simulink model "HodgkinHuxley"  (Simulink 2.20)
settings: Solver=ode45  StartTime=0.0  StopTime=1000  MaxStep=0.1  RelTol=1e-3  AbsTol=1e-6
undefined symbols (not defined in the file or in its folder): sfuny, sfunyst

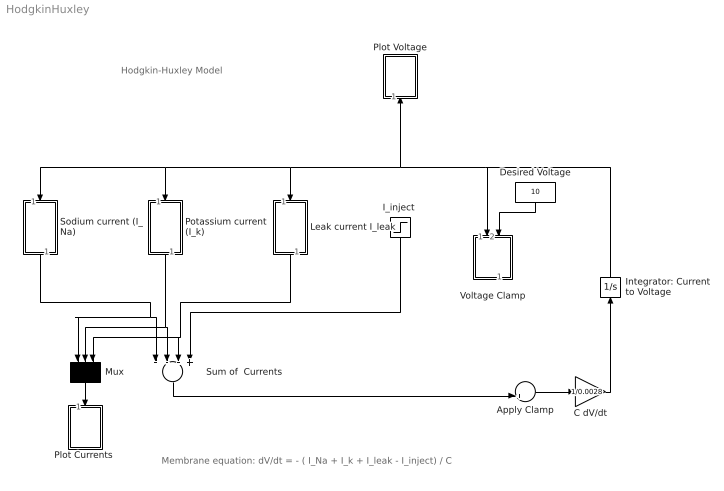
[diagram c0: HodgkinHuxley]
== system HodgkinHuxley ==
  note: Membrane equation: dV/dt = - ( I_Na + I_k + I_leak - I_inject) / C
  note: Hodgkin-Huxley Model
  Apply Clamp : Sum  Inputs=-+
  C dV/dt : Gain  Gain=1/0.0028
  Desired Voltage : Constant  Orientation=down  Value=10
  "I_inject " : Step  Orientation=down  Time=10  Before=0  After=.8
  Integrator: Current to Voltage : Integrator  Orientation=up  ExternalReset=none  InitialConditionSource=internal  InitialCondition=0  LimitOutput=off  UpperSaturationLimit=inf  LowerSaturationLimit=-inf  ShowSaturationPort=off  ShowStatePort=off  AbsoluteTolerance=auto
  Leak current I_leak : Subsystem  Orientation=down
  Mux : Mux  Orientation=down  Inputs=3
  "Plot Currents " : Subsystem  Orientation=down  mask(Storage scope.){}
      mask help: Storage scope using MATLAB graph window. Enter plotting ranges and line type.
      mask init:
      | npts = @4; color = @5; ax = [0, @1, @2, @3]; dt=-1;
  Plot Voltage : Subsystem  Orientation=up  LoadFcn=sfuny([],[],[],'LoadBlock')  StartFcn=sfuny([],[],[],'Start')  StopFcn=sfuny([],[],[],'Stop')  mask(Graph scope.){}
      mask help: Graph scope using MATLAB graph window. Enter plotting ranges and line type.
      mask init:
      | color = @4; ax = [0, @1, @2, @3]; dt = -1;
  Potassium current (I_k) : Subsystem  Orientation=down
  Sodium current (I_Na) : Subsystem  Orientation=down
  Sum of  Currents : Sum  Orientation=down  Inputs=---+
  Voltage Clamp : Subsystem  Orientation=down
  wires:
  Sum of  Currents/1 -> Apply Clamp/2
  Apply Clamp/1 -> C dV/dt/1
  Sodium current (I_Na)/1(I_Na) -> Mux/1, Sum of  Currents/1
  Potassium current (I_k)/1(output Ik) -> Mux/2, Sum of  Currents/2
  Leak current I_leak/1(output  I_leak) -> Mux/3, Sum of  Currents/3
  Mux/1 -> "Plot Currents "/1(x)
  Integrator: Current to Voltage/1 -> Plot Voltage/1(x), Potassium current (I_k)/1(input V), Sodium current (I_Na)/1(input V), Leak current I_leak/1(input V), Voltage Clamp/1(in_1)
  "I_inject "/1 -> Sum of  Currents/4
  Desired Voltage/1 -> Voltage Clamp/2(in_2)
  C dV/dt/1 -> Integrator: Current to Voltage/1

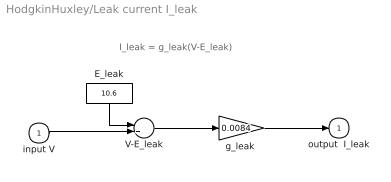
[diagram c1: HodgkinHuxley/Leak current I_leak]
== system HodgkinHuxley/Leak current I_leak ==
  note: I_leak = g_leak(V-E_leak)
  input V : Inport  Port=1  PortWidth=-1  SampleTime=-1
  E_leak : Constant  Orientation=down  Value=10.6
  V-E_leak : Sum  Inputs=-+
  "g_leak " : Gain  Gain=0.0084
  output  I_leak : Outport  Port=1  InitialOutput=0
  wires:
  "g_leak "/1 -> output  I_leak/1
  input V/1 -> V-E_leak/2
  E_leak/1 -> V-E_leak/1
  V-E_leak/1 -> "g_leak "/1

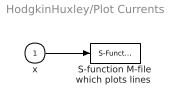
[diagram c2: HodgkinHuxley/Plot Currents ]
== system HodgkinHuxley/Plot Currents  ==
  x : Inport  Port=1  PortWidth=-1  SampleTime=-1
  "S-function M-file which plots lines " : S-Function  LoadFcn=sfunyst([],[],[],'LoadBlock')  FunctionName=sfunyst  Parameters=ax, color, npts, dt  PortCounts=[]  SFunctionModules=''
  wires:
  x/1 -> "S-function M-file which plots lines "/1

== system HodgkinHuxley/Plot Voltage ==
  x : Inport  Port=1  PortWidth=-1  SampleTime=-1
  "S-function M-file which plots lines " : S-Function  FunctionName=sfuny  Parameters=ax, color,dt  PortCounts=[]  SFunctionModules=''
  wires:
  x/1 -> "S-function M-file which plots lines "/1

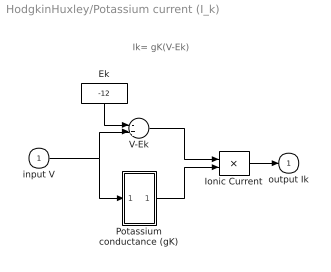
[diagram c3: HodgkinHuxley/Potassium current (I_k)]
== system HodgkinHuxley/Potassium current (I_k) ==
  note: Ik= gK(V-Ek)
  input V : Inport  Port=1  PortWidth=-1  SampleTime=-1
  Ek : Constant  Orientation=down  Value=-12
  Ionic Current : Product  Inputs=2
  Potassium conductance (gK) : Subsystem
  V-Ek : Sum  Inputs=-+
  output Ik : Outport  Port=1  InitialOutput=0
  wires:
  input V/1 -> Potassium conductance (gK)/1(input V), V-Ek/2
  Ionic Current/1 -> output Ik/1
  Ek/1 -> V-Ek/1
  V-Ek/1 -> Ionic Current/1
  Potassium conductance (gK)/1(output gK) -> Ionic Current/2

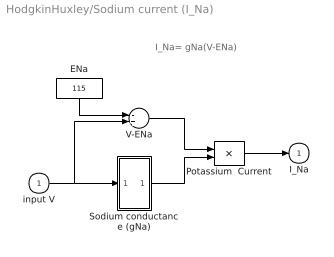
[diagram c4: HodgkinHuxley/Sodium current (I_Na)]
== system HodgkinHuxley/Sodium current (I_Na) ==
  note: I_Na= gNa(V-ENa)
  input V : Inport  Port=1  PortWidth=-1  SampleTime=-1
  ENa : Constant  Orientation=down  Value=115
  Potassium  Current : Product  Inputs=2
  Sodium conductance (gNa) : Subsystem
  V-ENa : Sum  Inputs=-+
  I_Na : Outport  Port=1  InitialOutput=0
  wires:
  input V/1 -> V-ENa/2, Sodium conductance (gNa)/1(input V)
  Potassium  Current/1 -> I_Na/1
  ENa/1 -> V-ENa/1
  V-ENa/1 -> Potassium  Current/1
  Sodium conductance (gNa)/1(ouput gNa) -> Potassium  Current/2

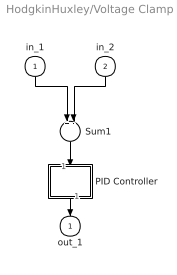
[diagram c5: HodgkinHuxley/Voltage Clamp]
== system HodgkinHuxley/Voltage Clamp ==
  in_1 : Inport  Orientation=down  Port=1  PortWidth=-1  SampleTime=-1
  in_2 : Inport  Orientation=down  Port=2  PortWidth=-1  SampleTime=-1
  PID Controller : Subsystem  Orientation=down  mask(PID Controller){}
      mask help: Enter expressions for proportional, integral, and derivative terms. P+I/s+Ds
      mask init:
      | P=@1; I=@2; D=@3;
  Sum1 : Sum  Orientation=down  Inputs=+-
  out_1 : Outport  Orientation=down  Port=1  InitialOutput=0
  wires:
  PID Controller/1(Out_1) -> out_1/1
  in_2/1 -> Sum1/2
  in_1/1 -> Sum1/1
  Sum1/1 -> PID Controller/1(In_1)

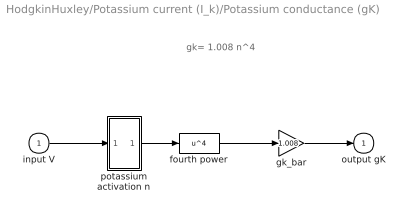
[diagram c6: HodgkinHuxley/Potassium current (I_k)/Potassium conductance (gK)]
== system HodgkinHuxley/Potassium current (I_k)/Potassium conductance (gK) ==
  note: gk= 1.008 n^4
  input V : Inport  Port=1  PortWidth=-1  SampleTime=-1
  fourth power : Fcn  Expr=u^4
  gk_bar : Gain  Gain=1.008
  potassium activation n : Subsystem
  output gK : Outport  Port=1  InitialOutput=0
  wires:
  input V/1 -> potassium activation n/1(input V)
  potassium activation n/1(output n) -> fourth power/1
  fourth power/1 -> gk_bar/1
  gk_bar/1 -> output gK/1

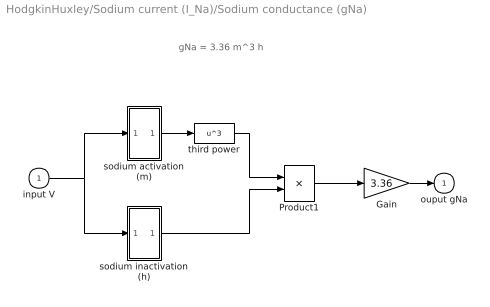
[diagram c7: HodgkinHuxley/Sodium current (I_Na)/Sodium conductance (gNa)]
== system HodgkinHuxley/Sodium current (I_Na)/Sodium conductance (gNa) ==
  note: gNa = 3.36 m^3 h
  input V : Inport  Port=1  PortWidth=-1  SampleTime=-1
  Gain : Gain  Gain=3.36
  Product1 : Product  Inputs=2
  sodium activation (m) : Subsystem
  sodium inactivation (h) : Subsystem
  third power : Fcn  Expr=u^3
  ouput gNa : Outport  Port=1  InitialOutput=0
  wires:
  Gain/1 -> ouput gNa/1
  Product1/1 -> Gain/1
  sodium inactivation (h)/1(output h) -> Product1/2
  third power/1 -> Product1/1
  input V/1 -> sodium activation (m)/1(input V), sodium inactivation (h)/1(input V)
  sodium activation (m)/1(output m) -> third power/1

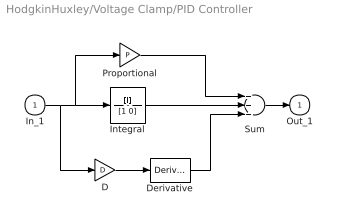
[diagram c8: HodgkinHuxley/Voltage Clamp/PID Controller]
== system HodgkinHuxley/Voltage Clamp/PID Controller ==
  In_1 : Inport  Port=1  PortWidth=-1  SampleTime=-1
  D : Gain  Gain=D
  Derivative : Derivative
  Integral : TransferFcn  Numerator=[I]  Denominator=[1 0]
  Proportional : Gain  Gain=P
  Sum : Sum  Inputs=+++
  Out_1 : Outport  Port=1  InitialOutput=0
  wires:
  Proportional/1 -> Sum/1
  Integral/1 -> Sum/2
  Derivative/1 -> Sum/3
  In_1/1 -> Proportional/1, Integral/1, D/1
  Sum/1 -> Out_1/1
  D/1 -> Derivative/1

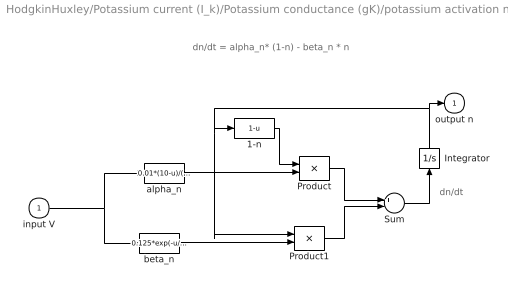
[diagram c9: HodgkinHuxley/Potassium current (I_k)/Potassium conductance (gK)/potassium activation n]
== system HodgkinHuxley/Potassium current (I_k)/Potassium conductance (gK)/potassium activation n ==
  note: dn/dt
  note: dn/dt = alpha_n* (1-n) - beta_n * n
  input V : Inport  Port=1  PortWidth=-1  SampleTime=-1
  1-n : Fcn  Expr=1-u
  Integrator : Integrator  Orientation=up  ExternalReset=none  InitialConditionSource=internal  InitialCondition=0.3117  LimitOutput=off  UpperSaturationLimit=inf  LowerSaturationLimit=-inf  ShowSaturationPort=off  ShowStatePort=off  AbsoluteTolerance=auto
  Product : Product  Inputs=2
  Product1 : Product  Inputs=2
  Sum : Sum  Inputs=+-
  alpha_n : Fcn  Expr=0.01*(10-u)/(exp(1-u/10)-1)
  beta_n : Fcn  Expr=0.125*exp(-u/80)
  output n : Outport  Port=1  InitialOutput=0
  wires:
  Integrator/1 -> Product1/1, 1-n/1, output n/1
  Sum/1 -> Integrator/1
  1-n/1 -> Product/1
  input V/1 -> alpha_n/1, beta_n/1
  alpha_n/1 -> Product/2
  beta_n/1 -> Product1/2
  Product1/1 -> Sum/2
  Product/1 -> Sum/1

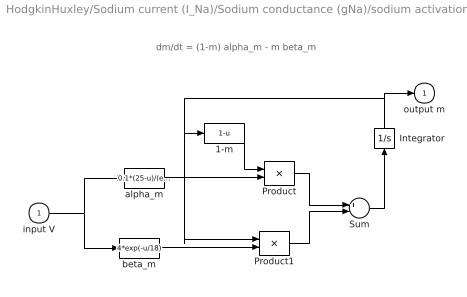
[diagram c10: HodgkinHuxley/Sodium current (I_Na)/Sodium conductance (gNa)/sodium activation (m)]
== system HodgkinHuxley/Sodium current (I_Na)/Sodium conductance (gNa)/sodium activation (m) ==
  note: dm/dt = (1-m) alpha_m - m beta_m
  input V : Inport  Port=1  PortWidth=-1  SampleTime=-1
  1-m : Fcn  Expr=1-u
  Integrator : Integrator  Orientation=up  ExternalReset=none  InitialConditionSource=internal  InitialCondition=0.0529  LimitOutput=off  UpperSaturationLimit=inf  LowerSaturationLimit=-inf  ShowSaturationPort=off  ShowStatePort=off  AbsoluteTolerance=auto
  Product : Product  Inputs=2
  Product1 : Product  Inputs=2
  Sum : Sum  Inputs=+-
  alpha_m : Fcn  Expr=0.1*(25-u)/(exp(2.5-u/10)-1)
  beta_m : Fcn  Expr=4*exp(-u/18)
  output m : Outport  Port=1  InitialOutput=0
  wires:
  Integrator/1 -> Product1/1, 1-m/1, output m/1
  input V/1 -> alpha_m/1, beta_m/1
  alpha_m/1 -> Product/2
  beta_m/1 -> Product1/2
  1-m/1 -> Product/1
  Product1/1 -> Sum/2
  Product/1 -> Sum/1
  Sum/1 -> Integrator/1

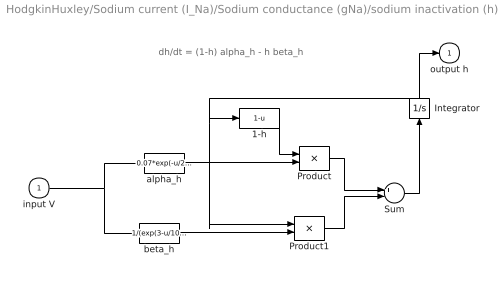
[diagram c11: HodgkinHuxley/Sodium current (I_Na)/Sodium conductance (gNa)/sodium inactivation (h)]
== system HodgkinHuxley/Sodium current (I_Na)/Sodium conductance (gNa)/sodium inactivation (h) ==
  note: dh/dt = (1-h) alpha_h - h beta_h
  input V : Inport  Port=1  PortWidth=-1  SampleTime=-1
  1-h : Fcn  Expr=1-u
  Integrator : Integrator  Orientation=up  ExternalReset=none  InitialConditionSource=internal  InitialCondition=0.5961  LimitOutput=off  UpperSaturationLimit=inf  LowerSaturationLimit=-inf  ShowSaturationPort=off  ShowStatePort=off  AbsoluteTolerance=auto
  Product : Product  Inputs=2
  Product1 : Product  Inputs=2
  Sum : Sum  Inputs=+-
  alpha_h : Fcn  Expr=0.07*exp(-u/20)
  beta_h : Fcn  Expr=1/(exp(3-u/10)+1)
  output h : Outport  Port=1  InitialOutput=0
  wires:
  Integrator/1 -> output h/1, 1-h/1, Product1/1
  input V/1 -> alpha_h/1, beta_h/1
  alpha_h/1 -> Product/2
  beta_h/1 -> Product1/2
  1-h/1 -> Product/1
  Product1/1 -> Sum/2
  Product/1 -> Sum/1
  Sum/1 -> Integrator/1
